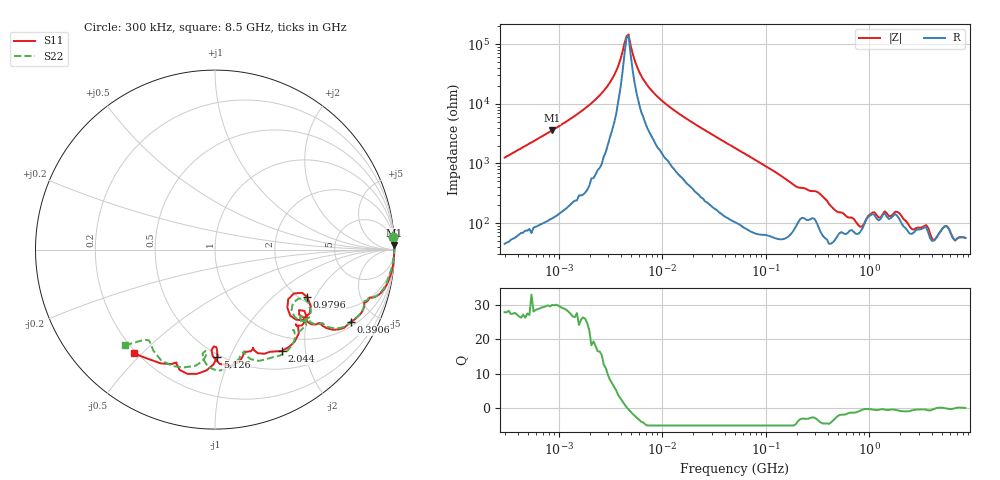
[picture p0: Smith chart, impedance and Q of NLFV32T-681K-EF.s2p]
! S-parameter Generated by TDK Corporation
! Copyright(C) 2015 TDK Corporation.
! All Rights Reserved.
! TDK P/N: NLFV32T-681K-EF (Inductors)
! Property: L=680uH at 796kHz
! Size(LxWxT): 3.2x2.5x2.2mm, 0.126x0.098x0.087inches
! Model Type: s2p (Touchstone File Format Version 1.0)
! Frequency: DC=Yes Start=0.3MHz Stop=8500MHz 225points Log-sweep
! Note:
! Model Generated on Jun. 23, 2015
! Hash(MD5):
! Port Assignments:
!  1 ---@@@--- 2
! Applicable Conditions:
!  Temperature = 25 degC
!  DC Bias Current = 0 A
!  Small Signal Operation
! Terms and conditions regarding TDK Simulation Models
! (1)This simulation model is being provided solely for informational purposes. Please refer to the specifications of the products in terms of detailed characteristics of such products.
! (2)In no event shall TDK Corporation of any of its subsidiaries be liable for any loss or damage arising, directly or indirectly,
!  From any information contained in this simulation model, including, but not limited to loss or damages arising from any inaccuracies, omissions or errors in connection with such information.
! (3)Any and all copyrights on this simulation model are owned by TDK Corporation.
!  Duplication or redistribution of this simulation model without prior written permission from TDK Corporation is prohibited.
! (4)This simulation model is subject to any modification or change without any prior notice.
! (5)Neither TDK Corporation nor any of its subsidiaries shall make any warranty, express or implied,
!  Including but not limited to the correctness, implied warranties of merchantability and fitness for a particular purpose with respect to this simulation models.
! (6)The use of this simulation model shall be deemed to have consented to the terms and conditions hereof.
# MHz S MA R 50
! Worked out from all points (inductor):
!   224 points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, 300 kHz to 8.5 GHz, reference 50 ohm
!   read as one part in series: L = 657 uH near 314.1 kHz
!   highest Q = 29.8 at 863.6 kHz (marker M1), where L = 661 uH
!   self-resonance near 4.519 MHz
!   S11 on the Smith chart (normalised r, x): 300 kHz: 2, +27; 390.6 MHz: 1.19, -3.63; 979.6 MHz: 2.17, -1.72; 2.044 GHz: 0.76, -1.59; 5.126 GHz: 0.48, -0.90; 8.5 GHz: 0.19, -0.47
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0.3  0.9944 4.2  0.07929 -83.8  0.08029 -84.0  0.9937 4.2
0.8636283  0.9984 1.5  0.02782 -86.7  0.02796 -87.0  0.9984 1.4
1.72111  0.9992 0.6  0.01263 -87.2  0.01268 -87.6  0.9996 0.5
3.275859  0.9994 0.1  0.003837 -82.1  0.003849 -82.4  0.9996 -0.0
4.732045  0.9994 -0.1  0.0006879 21.4  0.0006843 20.8  0.9993 -0.3
5.954923  0.9991 -0.3  0.002848 72.7  0.002841 72.5  0.9992 -0.4
9.430415  0.9989 -0.7  0.008171 81.3  0.008173 81.1  0.9988 -0.8
51.67171  0.9962 -4.3  0.05604 82.4  0.05606 82.2  0.9934 -4.4
187.1913  0.9364 -16.1  0.2137 63.9  0.2139 63.6  0.9358 -16.0
283.1228  0.8817 -19.6  0.2516 50.2  0.2519 50.0  0.8764 -19.3
390.6008  0.8575 -28.1  0.3484 49.8  0.3487 49.5  0.8592 -27.5
815.0429  0.5175 -38.8  0.5386 4.9  0.5393 4.7  0.5434 -38.3
979.5854  0.5774 -27.2  0.4172 -7.6  0.4169 -8.0  0.6023 -29.8
1551.304  0.6233 -43.0  0.4054 -8.3  0.4059 -8.8  0.6323 -45.8
2044.041  0.6773 -56.5  0.3898 -7.0  0.3904 -7.2  0.6928 -58.4
2572.272  0.5989 -68.9  0.4793 -19.0  0.4801 -19.5  0.6153 -73.7
3548.748  0.6277 -76.5  0.4019 -34.5  0.4029 -35.0  0.6686 -83.2
4073.536  0.594 -91.2  0.4875 -38.8  0.4902 -39.6  0.614 -96.1
5126.239  0.5976 -88.7  0.384 -65.1  0.3838 -65.5  0.6251 -96.4
6161.135  0.709 -102.6  0.3439 -61.1  0.3411 -61.3  0.6854 -116.1
7404.957  0.6811 -110.6  0.3347 -81.0  0.3357 -81.6  0.635 -127.6
8500  0.7333 -128.0  0.2557 -89.6  0.2555 -88.9  0.731 -133.4
